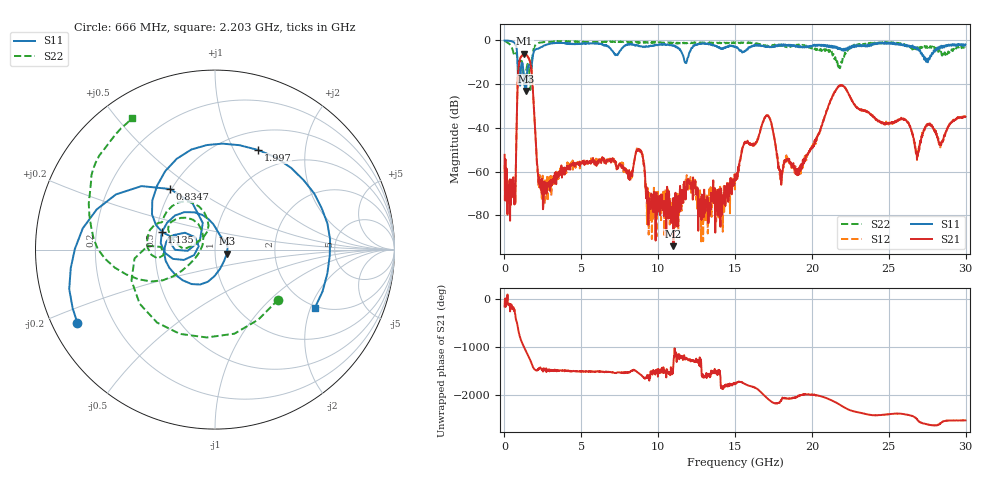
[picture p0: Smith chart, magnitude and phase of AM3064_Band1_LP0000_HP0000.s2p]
# Hz S DB R 50.0
!freq dBS11 angS11 dBS21 angS21 dBS12 angS12 dBS22 angS22
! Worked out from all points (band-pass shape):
!   1600 points, 10 MHz to 29.98 GHz, reference 50 ohm
!   highest |S21| = -6.10 dB at 1.303 GHz (marker M1); lowest = -94.1 dB at 10.99 GHz (marker M2)
!   |S21| within 3 dB of the highest: 990.4 MHz to 1.632 GHz (642 MHz wide, 49 % of centre)
!   lowest |S11| = -23.1 dB at 1.397 GHz (marker M3), VSWR 1.15, Z = 57 - j2.54 ohm
!   |S11| at or under -10 dB: 848.6 MHz to 1.795 GHz (946.1 MHz wide, 71.6 % of centre); 11.74 GHz to 11.84 GHz (105.5 MHz wide, 0.895 % of centre)
!   |S22| runs from -22.7 to -0.2 dB; largest |S21 - S12| = 0.0074
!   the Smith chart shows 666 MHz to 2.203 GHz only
!   S11 on the Smith chart (normalised r, x): 666 MHz: 0.07, -0.25; 834.7 MHz: 0.49, +0.40; 1.135 GHz: 0.53, +0.11; 1.997 GHz: 0.72, +1.25; 2.203 GHz: 1.94, -2.15
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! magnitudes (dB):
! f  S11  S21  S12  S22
! 10 MHz  0.0  -52.3  -56.9  -0.2
! 666 MHz  -1.2  -67.4  -68.5  -6.9
! 834.7 MHz  -7.5  -25.4  -25.3  -8.5
! 1.135 GHz  -10.1  -7.1  -7.1  -9.6
! 1.303 GHz  -20.3  -6.1  -6.0  -20.1
! 1.397 GHz  -23.1  -6.4  -6.3  -14.5
! 1.716 GHz  -12.7  -11.4  -11.4  -18.2
! 1.997 GHz  -4.4  -41.2  -41.3  -2.3
! 2.203 GHz  -3.8  -63.5  -65.8  -1.2
! 5.015 GHz  -1.4  -56.2  -55.3  -0.6
! 8.763 GHz  -2.7  -50.1  -50.6  -1.1
! 9.401 GHz  -2.5  -72.2  -70.7  -0.8
! 10 GHz  -2.0  -77.8  -71.5  -0.9
! 10.99 GHz  -2.5  -94.1  -80.7  -1.2
! 15 GHz  -3.0  -63.9  -62.3  -1.4
! 17.05 GHz  -2.9  -34.5  -34.1  -2.7
! 17.95 GHz  -2.3  -61.9  -63.3  -2.0
! 19.99 GHz  -2.8  -48.8  -48.4  -3.5
! 21.83 GHz  -3.7  -20.8  -20.6  -12.7
! 25 GHz  -1.0  -37.8  -37.8  -1.1
! 26.85 GHz  -4.3  -51.2  -52.6  -3.1
! 29.98 GHz  -1.8  -35.0  -34.9  -3.2
